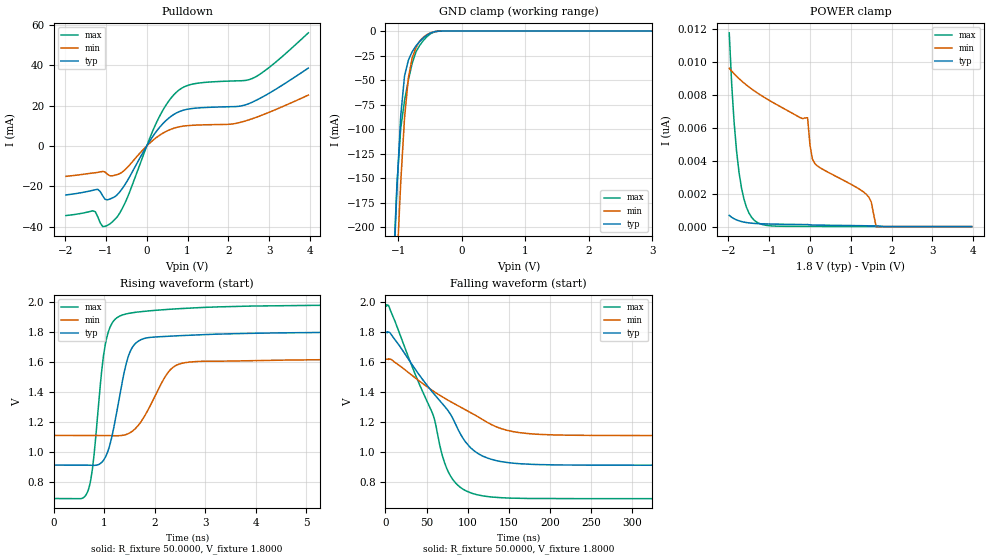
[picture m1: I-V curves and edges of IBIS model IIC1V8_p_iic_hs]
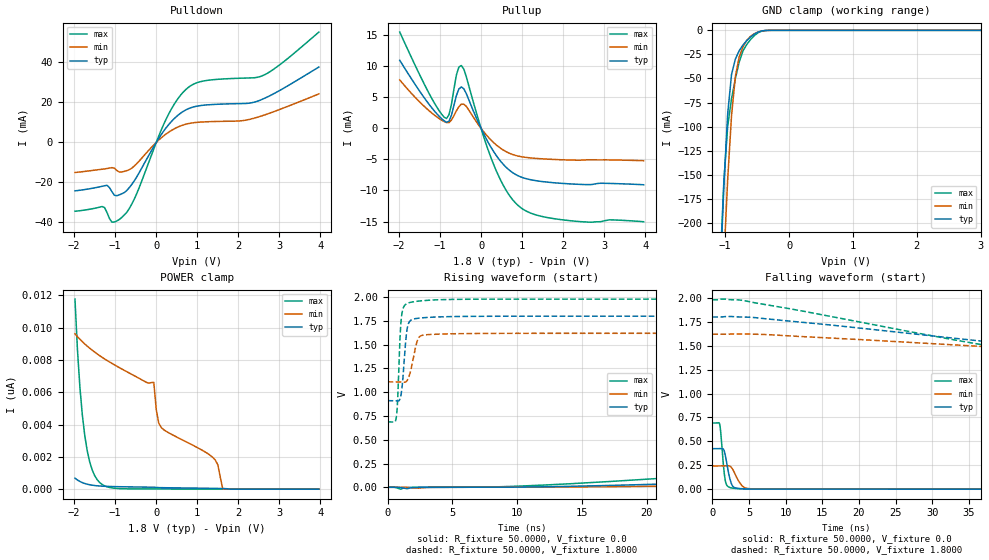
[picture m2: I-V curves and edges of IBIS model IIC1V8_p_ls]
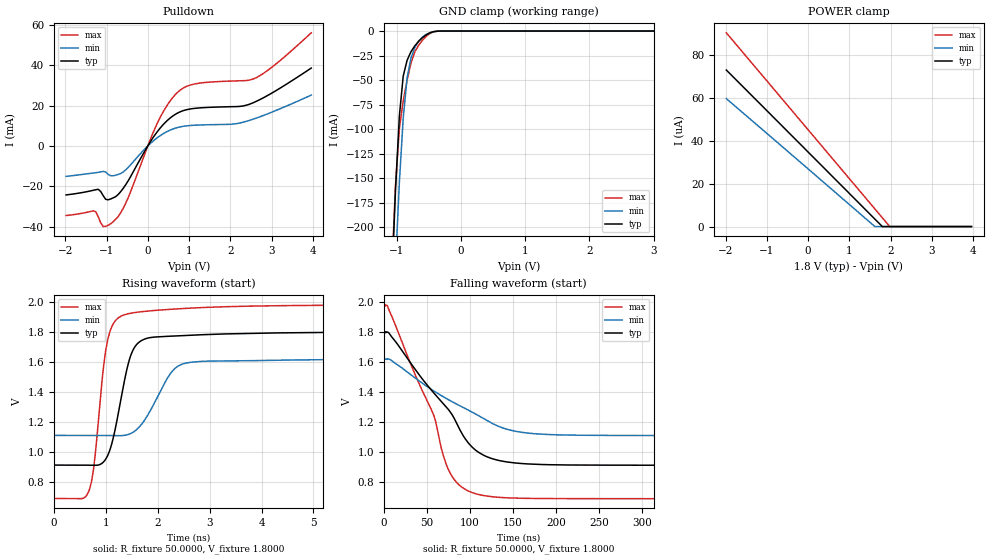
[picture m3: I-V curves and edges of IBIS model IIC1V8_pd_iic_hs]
| IBIS file qfp64afe_1p8v.ibs generated by Viper version: 2020.12.17
[IBIS Ver]   5.0
[Comment Char]   |_char
[File Name]   qfp64afe_1p8v.ibs
[File Rev]   1.3
[Date]   Thu Dec 17 17:50:21 2020
[Source]   NXP Viper 2020.12.17
[Notes]
[Disclaimer] IMPORTANT NOTICE
  This information is provided on an AS IS basis and without warranty.
  IN NO EVENT SHALL NXP BE LIABLE FOR INCIDENTAL OR CONSEQUENTIAL
  DAMAGES ARISING FROM USE OF THIS INFORMATION. THIS DISCLAIMER OF
  WARRANTY EXTENDS TO THE USER OF THE INFORMATION, AND TO THEIR CUSTOMERS
  OR USERS OF PRODUCTS  AND IS IN LIEU OF ALL WARRANTIES WHETHER EXPRESS,
  IMPLIED, OR STATUTORY, INCLUDING IMPLIED WARRANTIES OF MERCHANTABILITY
  OR FITNESS FOR PARTICULAR PURPOSE.
  NXP does not represent or warrant that the information furnished
  hereunder is free of infringement of any third party patents,
  copyrights, trade secrets, or other intellectual property rights.
  NXP does not represent or warrant that the information is free of
  defect, or that it meets any particular standard, requirements or need
  of the user of the infomation or their customers.
  NXP reserves the right to change the information in this file
  without notice.
   http://www.nxp.com
[Copyright]   (C) Copyright NXP 2004 - 2020, All Rights Reserved.
|   qfp64Afe
[Component]   qfp64Afe
[Manufacturer]   NXP
[Package]
| variable   typ   min   max
R_pkg   0.18002   0.098036   0.22836
L_pkg   3.270e-09   2.478e-09   3.882e-09
C_pkg   4.877e-13   4.194e-13   6.388e-13
[Pin] signal_name   model_name   R_pin   L_pin   C_pin
1   P2_1   gpio   0.20176   3.768e-09 4.934e-13
2   OPAMP2_INN   NC   0.18655   3.432e-09 5.614e-13
3   P0_1   gpio   0.1882   3.425e-09 5.543e-13
4   P1_0   gpio   0.18167   3.391e-09 4.852e-13
5   ADC1IN1B   NC   0.17508   3.272e-09 4.734e-13
6   ADC1IN1A   NC   0.17211   3.184e-09 4.709e-13
7   P0_11   gpio   0.17322   3.095e-09 4.516e-13
8   VDDA   POWER   NA   NA   NA
9   VREF_OUT   NC   0.098933  2.478e-09 5.107e-13
10   VREFP   NC   0.098036  2.682e-09 4.989e-13
11   VREFN   NC   0.10339   2.593e-09 5.200e-13
12   VSSA   GND   NA   NA   NA
13   P0_16   gpio   0.18219   3.272e-09 4.683e-13
14   P0_10   gpio   0.18473   3.372e-09 4.943e-13
15   P0_15   gpio   0.1948   3.518e-09 5.647e-13
16   P0_31   gpio   0.21166   3.882e-09 5.047e-13
17   P0_8   gpio   0.19981   3.690e-09 4.818e-13
18   OPAMP0_INN   NC   0.18485   3.354e-09 5.404e-13
19   P0_27   gpio   0.1771   3.251e-09 5.158e-13
20   OPAMP1_INN   NC   0.17264   3.242e-09 4.518e-13
21   XTAL32M_N   NC   0.17308   3.207e-09 4.514e-13
22   XTAL32M_P   NC   0.17099   3.143e-09 4.435e-13
23   RESETN   gpio   0.17312   3.058e-09 4.290e-13
24   VDD_CORE   POWER   NA   NA   NA
25   P1_22   gpio   0.17347   2.976e-09 4.359e-13
26   P0_17   gpio   0.17222   3.063e-09 4.368e-13
27   P0_7   gpio   0.17974   2.960e-09 4.541e-13
28   VDDE_2   POWER   NA   NA   NA
29   VSS_MAIN_PWR   GND   NA   NA   NA
30   VSS_MAIN   GND   NA   NA   NA
31   LX   NC   0.12471   2.527e-09 6.388e-13
32   VDD_MAIN_PWR   NC   NA   NA   NA
33   XTAL32K_P   NC   0.20305   3.722e-09 4.831e-13
34   XTAL32K_N   NC   0.18797   3.388e-09 5.425e-13
35   VBAT   NC   0.17937   3.272e-09 4.763e-13
36   P0_0   gpio   0.17575   3.216e-09 4.542e-13
37   P0_9   gpio   0.17142   3.151e-09 4.522e-13
38   P0_18   gpio   0.17027   3.108e-09 4.408e-13
39   P1_13   gpio   0.17092   3.083e-09 4.194e-13
40   P1_1   gpio   0.17351   3.079e-09 4.367e-13
41   P0_26   gpio   0.17937   3.140e-09 4.480e-13
42   P1_2   gpio   0.18924   3.260e-09 4.417e-13
43   P1_3   gpio   0.20575   3.278e-09 4.623e-13
44   VDDE_4   POWER   NA   NA   NA
45   P0_24   gpio   0.18768   3.277e-09 4.591e-13
46   P0_13   iic   0.19613   3.445e-09 5.506e-13
47   P0_14   iic   0.20782   3.616e-09 5.657e-13
48   P0_20   gpio   0.21594   3.876e-09 4.850e-13
49   P0_21   gpio   0.20723   3.837e-09 4.904e-13
50   P0_22   gpio   0.1962   3.547e-09 5.661e-13
51   P0_25   gpio   0.18792   3.420e-09 5.062e-13
52   P0_2   gpio   0.18663   3.397e-09 4.750e-13
53   P1_15   gpio   0.17882   3.273e-09 4.700e-13
54   P0_19   gpio   0.17446   3.156e-09 4.633e-13
55   P0_3   gpio   0.17673   3.008e-09 4.457e-13
56   VDDE_4   POWER   NA   NA   NA
57   P0_4   gpio   0.17637   3.003e-09 4.457e-13
58   P1_16   gpio   0.17537   3.170e-09 4.476e-13
59   P0_6   gpio   0.17935   3.248e-09 4.687e-13
60   P0_5   gpio   0.18758   3.378e-09 4.757e-13
61   P0_29   gpio   0.19171   3.430e-09 4.834e-13
62   P1_11   gpio   0.20582   3.539e-09 5.647e-13
63   P0_30   gpio   0.22836   3.428e-09 5.818e-13
64   VDDE_4   POWER   NA   NA   NA
65   VSS   GND   NA   NA   NA
[Pin Mapping]   pulldown_ref   pullup_ref
1   VSS   VDDA
2   NC   NC
3   VSS   VDDA
4   VSS   VDDA
5   NC   NC
6   NC   NC
7   VSS   VDDA
8   NC   VDDA
9   NC   NC
10   NC   NC
11   NC   NC
12   VSSA   NC
13   VSS   VDDA
14   VSS   VDDA
15   VSS   VDDA
16   VSS   VDDA
17   VSS   VDDA
18   NC   NC
19   VSS   VDDA
20   NC   NC
21   NC   NC
22   NC   NC
23   VSS   VDDE_2
24   NC   VDD_CORE
25   VSS   VDDE_2
26   VSS   VDDE_2
27   VSS   VDDE_2
28   NC   VDDE_2
29   VSS_MAIN_PWR   NC
30   VSS_MAIN   NC
31   NC   NC
32   NC   NC
33   NC   NC
34   NC   NC
35   NC   NC
36   VSS   VDDE_4
37   VSS   VDDE_4
38   VSS   VDDE_4
39   VSS   VDDE_4
40   VSS   VDDE_4
41   VSS   VDDE_4
42   VSS   VDDE_4
43   VSS   VDDE_4
44   NC   VDDE_4
45   VSS   VDDE_4
46   VSS   VDDE_4
47   VSS   VDDE_4
48   VSS   VDDE_4
49   VSS   VDDE_4
50   VSS   VDDE_4
51   VSS   VDDE_4
52   VSS   VDDE_4
53   VSS   VDDE_4
54   VSS   VDDE_4
55   VSS   VDDE_4
56   NC   VDDE_4
57   VSS   VDDE_4
58   VSS   VDDE_4
59   VSS   VDDE_4
60   VSS   VDDE_4
61   VSS   VDDE_4
62   VSS   VDDE_4
63   VSS   VDDE_4
64   NC   VDDE_4
65   VSS   NC
|*   Model Selector   *
[Model Selector] gpio
MFIO1V8_pd_hs   EPUN=1 EPD=1 EHS=1
MFIO1V8_pd_ls   EPUN=1 EPD=1 EHS=0
MFIO1V8_pu_hs   EPUN=0 EPD=0 EHS=1
MFIO1V8_pu_ls   EPUN=0 EPD=0 EHS=0
MFIO1V8_p_hs   EPUN=1 EPD=0 EHS=1
MFIO1V8_p_ls   EPUN=1 EPD=0 EHS=0
MFIO1V8_r_hs   EPUN=0 EPD=1 EHS=1
MFIO1V8_r_ls   EPUN=0 EPD=1 EHS=0
[Model Selector] iic
IIC1V8_pd_hs   EGP=1 EPUN=1 EPD=1 EHS=1
IIC1V8_pd_ls   EGP=1 EPUN=1 EPD=1 EHS=0
IIC1V8_p_hs   EGP=1 EPUN=1 EPD=0 EHS=1
IIC1V8_p_ls   EGP=1 EPUN=1 EPD=0 EHS=0
IIC1V8_pu_hs   EGP=1 EPUN=0 EPD=0 EHS=1
IIC1V8_pu_ls   EGP=1 EPUN=0 EPD=0 EHS=0
IIC1V8_r_hs   EGP=1 EPUN=0 EPD=1 EHS=1
IIC1V8_r_ls   EGP=1 EPUN=0 EPD=1 EHS=0
IIC1V8_pd_iic_hs   EGP=0 ECS=0 EPUN=1 EPD=1
IIC1V8_p_iic_hs   EGP=0 ECS=0 EPUN=1 EPD=0
IIC1V8_pu_iic_hs   EGP=0 ECS=0 EPUN=0 EPD=0
IIC1V8_r_iic_hs   EGP=0 ECS=0 EPUN=0 EPD=1
IIC1V8_pd_iic_pu_hs   EGP=0 ECS=1 EPUN=1 EPD=1 SSEL=1
IIC1V8_p_iic_pu_hs   EGP=0 ECS=1 EPUN=1 EPD=0 SSEL=1
IIC1V8_pu_iic_pu_hs   EGP=0 ECS=1 EPUN=0 EPD=0 SSEL=1
IIC1V8_r_iic_pu_hs   EGP=0 ECS=1 EPUN=0 EPD=1 SSEL=1
| End [Component] qfp64Afe
| Models and submodels in the file (24): IIC1V8_p_hs (I/O), IIC1V8_p_iic_hs (I/O_open_drain), IIC1V8_p_iic_pu_hs (I/O_open_drain), IIC1V8_p_ls (I/O), IIC1V8_pd_hs (I/O), IIC1V8_pd_iic_hs (I/O_open_drain), IIC1V8_pd_iic_pu_hs (I/O_open_drain), IIC1V8_pd_ls (I/O), IIC1V8_pu_hs (I/O), IIC1V8_pu_iic_hs (I/O_open_drain), IIC1V8_pu_iic_pu_hs (I/O_open_drain), IIC1V8_pu_ls (I/O), IIC1V8_r_hs (I/O), IIC1V8_r_iic_hs (I/O_open_drain), IIC1V8_r_iic_pu_hs (I/O_open_drain), IIC1V8_r_ls (I/O), MFIO1V8_p_hs (I/O), MFIO1V8_p_ls (I/O), MFIO1V8_pd_hs (I/O), MFIO1V8_pd_ls (I/O), MFIO1V8_pu_hs (I/O), MFIO1V8_pu_ls (I/O), MFIO1V8_r_hs (I/O), MFIO1V8_r_ls (I/O)
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[Model] IIC1V8_p_iic_hs
|   Model IIC1V8_p_iic_hs
| This model was characterised for following simulation conditions:
| External (pad) voltage:
|   - Typ: 1.8V,   - Min: 1.62V,   - Max: 1.98V
| Library cells for typ/min/max conditions are connected as defined below:
|  IO - External Pad
|  A - Core Input
|  EN - Output Buffer Enable
|  BOOST - vdde
|  ECS - gnd
|  EGP - gnd
|  ENZI - vdd
|  EPD - gnd
|  EPUN - vdd
|  ZI - NC
|  ZIF - NC
|  gnd - gnd
|  gnde - gnde
|  vdd - vdd
|  vdde - vdde
| All other pins connected to ground
Model_type I/O_open_drain
Polarity   Non-Inverting
Enable   Active-Low
Vinl =   0.5400V
Vinh =   1.2600V
Vmeas =  0.9000V
Cref =   0.0F
Rref =   1000.000
Vref =   1.8000V
C_comp   3.6454pF   3.5038pF   3.7808pF
|C_comp_pullup   0.9524pF   0.9269pF   0.9624pF
|C_comp_pulldown   2.3410pF   2.4924pF   2.1971pF
[Model Spec]
| variable   typ   min   max
Vinh   0.5400V   0.4860V   0.5940V
Vinl   1.2600V   1.1340V   1.3860V
Vmeas   0.9000V   0.8100V   0.9900V
Vref   1.8000V   1.6200V   1.9800V
Cref   0.0F   0.0F   0.0F
Rref   1.0000k   1.0000k   1.0000k
[Temperature Range]   25.0000   0.1250k   -40.0000
[Voltage Range]   1.8000V   1.6200V   1.9800V
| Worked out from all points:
|   slope of the pulldown table from 0 to 0.27 V, typ, clamps not added: 33.4 ohm
|   GND clamp passes 1 mA (typ) near -0.44 V on its own axis
|   rising waveform, R_fixture 50.0000, V_fixture 1.8000: 20-80 % time 321ps typ, 491ps min, 237ps max; typ from 0.911 V to 1.8 V
|   falling waveform, R_fixture 50.0000, V_fixture 1.8000: 20-80 % time 66.9ns typ, 88.7ns min, 48.9ns max; typ from 1.8 V to 0.911 V
[Pulldown]
|Voltage   I(typ)   I(min)   I(max)
-1.98V    -24.22mA   -15.04mA   -34.42mA
-1.32V    -21.94mA   -13.4mA    -32.06mA
-1.2V     -21.45mA   -13.05mA   -35.06mA
-1.08V    -24.63mA   -12.6mA    -39.9mA
-900mV    -26.23mA   -14.78mA   -38.53mA
-540mV    -19.33mA   -11.9mA    -28.53mA
300mV     8.856mA    5.096mA    14.12mA
720mV     16.26mA    9.117mA    26.48mA
1.14V     18.6mA     10.26mA    30.69mA
2.1V      19.45mA    10.9mA     32.16mA
2.58V     21.61mA    13.44mA    33.34mA
3.96V     38.56mA    25.19mA    55.99mA
[GND_clamp]
|Voltage   I(typ)   I(min)   I(max)
-1.98V    -2.104A    -2.075A    -2.136A
-1.08V    -259.3mA   -333mA     -246.9mA
-1.02V    -161.8mA   -238.7mA   -157.1mA
-960mV    -86.74mA   -154.7mA   -99.46mA
-900mV    -45.95mA   -88.82mA   -71.05mA
-840mV    -29.9mA    -47.99mA   -50.25mA
-780mV    -21.15mA   -27.64mA   -32.98mA
-720mV    -15.16mA   -16.87mA   -21.26mA
-660mV    -10.56mA   -10.24mA   -14.56mA
-540mV    -3.788mA   -3.398mA   -5.292mA
-300mV    -15.94uA   -36uA      -16.34uA
3.96V     0A         0A         0A
[POWER_clamp]
|Voltage   I(typ)   I(min)   I(max)
-1.98V    679.6pA    9.61nA     11.76nA
-1.86V    475.2pA    9.277nA    6.313nA
-1.74V    349.2pA    8.982nA    3.292nA
-1.56V    245.6pA    8.597nA    1.186nA
-1.32V    186pA      8.161nA    293.2pA
-60mV     124.8pA    6.606nA    14.31pA
0V        105.5pA    4.916nA    11.81pA
120mV     93.21pA    3.82nA     10.91pA
1.38V     50pA       1.96nA     2.877pA
1.5V      45.28pA    1.501nA    2.149pA
1.62V     39.18pA    0A         1.42pA
3.96V     0A         0A         0A
[Ramp]
| variable   typ   min   max
dV/dt_r  0.5334/0.3209n   0.3066/0.4909n   0.7753/0.2369n
dV/dt_f  0.5334/66.9323n   0.3066/88.7325n   0.7753/48.9497n
R_load = 50.0000
[Rising Waveform]
R_fixture= 50.0000
V_fixture= 1.8000
V_fixture_min= 1.6200
V_fixture_max= 1.9800
|time   V(typ)   V(min)   V(max)
0s        911mV      1.109V     687.8mV
683.3ps   910.2mV    1.109V     745.5mV
780.5ps   909.1mV    1.109V     927.7mV
1.017ns   961.1mV    1.108V     1.71V
1.277ns   1.32V      1.107V     1.9V
1.506ns   1.663V     1.126V     1.925V
1.797ns   1.757V     1.237V     1.938V
2.547ns   1.776V     1.591V     1.956V
6.124ns   1.798V     1.616V     1.979V
1us       1.8V       1.62V      1.98V
[Falling Waveform]
R_fixture= 50.0000
V_fixture= 1.8000
V_fixture_min= 1.6200
V_fixture_max= 1.9800
|time   V(typ)   V(min)   V(max)
0s        1.8V       1.62V      1.98V
4.033ns   1.8V       1.621V     1.975V
57.1ns    1.4V       1.41V      1.258V
68.97ns   1.323V     1.369V     978.6mV
76.93ns   1.269V     1.343V     860.5mV
95.01ns   1.085V     1.288V     749mV
110.3ns   997.3mV    1.242V     715.6mV
148.2ns   929.5mV    1.144V     692.6mV
208ns     913.4mV    1.113V     688.4mV
1us       911.1mV    1.109V     687.9mV
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[Model] IIC1V8_p_ls
|   Model IIC1V8_p_ls
| This model was characterised for following simulation conditions:
| External (pad) voltage:
|   - Typ: 1.8V,   - Min: 1.62V,   - Max: 1.98V
| Library cells for typ/min/max conditions are connected as defined below:
|  IO - External Pad
|  A - Core Input
|  EN - Output Buffer Enable
|  BOOST - vdde
|  EGP - vdd
|  EHS - gnd
|  ENZI - vdd
|  EPD - gnd
|  EPUN - vdd
|  ZI - NC
|  ZIF - NC
|  gnd - gnd
|  gnde - gnde
|  vdd - vdd
|  vdde - vdde
| All other pins connected to ground
Model_type I/O
Polarity   Non-Inverting
Enable   Active-Low
Vinl =   0.5400V
Vinh =   1.2600V
Vmeas =  0.9000V
Cref =   0.0F
Rref =   1.0000k
Vref =   0.0V
C_comp   3.6452pF   3.5037pF   3.7805pF
|C_comp_pullup   0.9521pF   0.9262pF   0.9623pF
|C_comp_pulldown   2.3411pF   2.4927pF   2.1971pF
[Model Spec]
| variable   typ   min   max
Vinh   0.5400V   0.4860V   0.5940V
Vinl   1.2600V   1.1340V   1.3860V
Vmeas   0.9000V   0.8100V   0.9900V
[Temperature Range]   25.0000   0.1250k   -40.0000
[Voltage Range]   1.8000V   1.6200V   1.9800V
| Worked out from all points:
|   slope of the pulldown table from 0 to 0.27 V, typ, clamps not added: 33.4 ohm
|   slope of the pullup table from 0 to 0.27 V, typ, clamps not added: 80.7 ohm
|   GND clamp passes 1 mA (typ) near -0.44 V on its own axis
|   rising waveform, R_fixture 50.0000, V_fixture 0.0: 20-80 % time 70.1ns typ, 82ns min, 57.1ns max; typ from 0 V to 0.423 V
|   rising waveform, R_fixture 50.0000, V_fixture 1.8000: 20-80 % time 319ps typ, 487ps min, 235ps max; typ from 0.911 V to 1.8 V
|   falling waveform, R_fixture 50.0000, V_fixture 0.0: 20-80 % time 672ps typ, 1.04ns min, 474ps max; typ from 0.423 V to 0 V
|   falling waveform, R_fixture 50.0000, V_fixture 1.8000: 20-80 % time 66.9ns typ, 88.7ns min, 49ns max; typ from 1.8 V to 0.911 V
[Pulldown]
|Voltage   I(typ)   I(min)   I(max)
-1.98V    -24.22mA   -15.04mA   -34.42mA
-1.32V    -21.94mA   -13.4mA    -32.06mA
-1.2V     -21.45mA   -13.05mA   -35.06mA
-1.08V    -24.63mA   -12.6mA    -39.9mA
-900mV    -26.23mA   -14.78mA   -38.53mA
-720mV    -24.07mA   -14.13mA   -34.99mA
-540mV    -19.33mA   -11.9mA    -28.53mA
300mV     8.856mA    5.096mA    14.12mA
720mV     16.26mA    9.117mA    26.48mA
1.14V     18.6mA     10.26mA    30.69mA
2.58V     21.56mA    13.35mA    33.32mA
3.96V     37.73mA    24.28mA    55.2mA
[Pullup]
|Voltage   I(typ)   I(min)   I(max)
-1.98V    10.95mA    7.799mA    15.5mA
-1.32V    4.346mA    3.159mA    6.304mA
-900mV    1.218mA    1.094mA    1.804mA
-780mV    1.156mA    929.2uA    2.224mA
-600mV    5.286mA    2.831mA    8.611mA
-480mV    6.667mA    3.906mA    10.12mA
-420mV    6.372mA    3.889mA    9.539mA
360mV     -4.265mA   -2.608mA   -6.666mA
660mV     -6.57mA    -3.917mA   -10.5mA
960mV     -7.8mA     -4.537mA   -12.74mA
2.04V     -8.889mA   -5.075mA   -14.77mA
3.96V     -9.081mA   -5.209mA   -15.04mA
[GND_clamp]
|Voltage   I(typ)   I(min)   I(max)
-1.98V    -2.104A    -2.075A    -2.136A
-1.08V    -259.3mA   -333mA     -246.9mA
-1.02V    -161.8mA   -238.7mA   -157.1mA
-960mV    -86.74mA   -154.7mA   -99.46mA
-900mV    -45.95mA   -88.82mA   -71.05mA
-840mV    -29.9mA    -47.99mA   -50.25mA
-780mV    -21.15mA   -27.64mA   -32.98mA
-720mV    -15.16mA   -16.87mA   -21.26mA
-660mV    -10.56mA   -10.24mA   -14.56mA
-540mV    -3.788mA   -3.398mA   -5.292mA
-300mV    -15.94uA   -36uA      -16.34uA
3.96V     0A         0A         0A
[POWER_clamp]
|Voltage   I(typ)   I(min)   I(max)
-1.98V    679.6pA    9.61nA     11.76nA
-1.86V    475.2pA    9.277nA    6.313nA
-1.74V    349.2pA    8.982nA    3.292nA
-1.56V    245.6pA    8.597nA    1.186nA
-1.32V    186pA      8.161nA    293.2pA
-60mV     124.8pA    6.606nA    14.31pA
0V        105.5pA    4.916nA    11.81pA
120mV     93.21pA    3.82nA     10.91pA
1.38V     50pA       1.96nA     2.877pA
1.5V      45.28pA    1.501nA    2.149pA
1.62V     39.18pA    0A         1.42pA
3.96V     0A         0A         0A
[Ramp]
| variable   typ   min   max
dV/dt_r  0.2539/70.1178n   0.1457/81.9302n   0.4150/57.0489n
dV/dt_f  0.5334/66.9358n   0.3066/88.6649n   0.7753/48.9538n
R_load = 50.0000
[Rising Waveform]
R_fixture= 50.0000
V_fixture= 0.0
V_fixture_min= 0.0
V_fixture_max= 0.0
|time   V(typ)   V(min)   V(max)
0s        602.8pV    52.95nV    41.9pV
1.012ns   -3.31mV    192.5uV    -19.98mV
1.632ns   -11.39mV   -2.738mV   -1.795mV
12.68ns   6.299mV    1.388mV    27.19mV
45.88ns   145.4mV    64.89mV    304.8mV
84.55ns   285.2mV    143.4mV    561.1mV
103.3ns   339.8mV    172mV      629.2mV
134ns     392.1mV    207.9mV    672.5mV
250.9ns   422.4mV    241.3mV    691.3mV
1us       423.2mV    242.8mV    691.7mV
[Rising Waveform]
R_fixture= 50.0000
V_fixture= 1.8000
V_fixture_min= 1.6200
V_fixture_max= 1.9800
|time   V(typ)   V(min)   V(max)
0s        911mV      1.109V     687.8mV
685.2ps   909.5mV    1.109V     745.1mV
787ps     907.1mV    1.109V     945.8mV
1.007ns   951.3mV    1.108V     1.694V
1.269ns   1.304V     1.105V     1.904V
1.479ns   1.639V     1.118V     1.932V
1.768ns   1.755V     1.218V     1.945V
2.476ns   1.78V      1.585V     1.96V
5.596ns   1.797V     1.616V     1.978V
1us       1.8V       1.62V      1.98V
[Falling Waveform]
R_fixture= 50.0000
V_fixture= 0.0
V_fixture_min= 0.0
V_fixture_max= 0.0
|time   V(typ)   V(min)   V(max)
0s        423.2mV    242.8mV    691.7mV
1.011ns   423.2mV    242.8mV    674.4mV
1.154ns   424.5mV    242.8mV    586.3mV
1.621ns   398.5mV    242.8mV    166.3mV
1.942ns   280.1mV    244.4mV    44.84mV
2.413ns   102.2mV    239.4mV    16.8mV
2.833ns   25.91mV    200.2mV    9.661mV
4.004ns   4.701mV    40.3mV     3.498mV
5.055ns   2.01mV     5.162mV    2.038mV
1us       19.02nV    85.51nV    10.92nV
[Falling Waveform]
R_fixture= 50.0000
V_fixture= 1.8000
V_fixture_min= 1.6200
V_fixture_max= 1.9800
|time   V(typ)   V(min)   V(max)
0s        1.8V       1.62V      1.98V
4.079ns   1.8V       1.623V     1.975V
57.22ns   1.399V     1.41V      1.256V
69.33ns   1.321V     1.367V     971.7mV
77.23ns   1.267V     1.342V     857.4mV
95.69ns   1.079V     1.287V     746.9mV
111ns     994.9mV    1.239V     714.6mV
149.1ns   928.8mV    1.143V     692.4mV
207.1ns   913.6mV    1.113V     688.4mV
1us       911.1mV    1.109V     687.9mV
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[Model] IIC1V8_pd_iic_hs
|   Model IIC1V8_pd_iic_hs
| This model was characterised for following simulation conditions:
| External (pad) voltage:
|   - Typ: 1.8V,   - Min: 1.62V,   - Max: 1.98V
| Library cells for typ/min/max conditions are connected as defined below:
|  IO - External Pad
|  A - Core Input
|  EN - Output Buffer Enable
|  BOOST - vdde
|  ECS - gnd
|  EGP - gnd
|  ENZI - vdd
|  EPD - vdd
|  EPUN - vdd
|  ZI - NC
|  ZIF - NC
|  gnd - gnd
|  gnde - gnde
|  vdd - vdd
|  vdde - vdde
| All other pins connected to ground
Model_type I/O_open_drain
Polarity   Non-Inverting
Enable   Active-Low
Vinl =   0.5400V
Vinh =   1.2600V
Vmeas =  0.9000V
Cref =   0.0F
Rref =   1000.000
Vref =   1.8000V
C_comp   3.6138pF   3.4666pF   3.7547pF
|C_comp_pullup   0.9378pF   0.9163pF   0.9441pF
|C_comp_pulldown   2.3253pF   2.4781pF   2.1797pF
[Model Spec]
| variable   typ   min   max
Vinh   0.5400V   0.4860V   0.5940V
Vinl   1.2600V   1.1340V   1.3860V
Vmeas   0.9000V   0.8100V   0.9900V
Vref   1.8000V   1.6200V   1.9800V
Cref   0.0F   0.0F   0.0F
Rref   1.0000k   1.0000k   1.0000k
[Temperature Range]   25.0000   0.1250k   -40.0000
[Voltage Range]   1.8000V   1.6200V   1.9800V
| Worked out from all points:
|   slope of the pulldown table from 0 to 0.27 V, typ, clamps not added: 33.4 ohm
|   GND clamp passes 1 mA (typ) near -0.44 V on its own axis
|   rising waveform, R_fixture 50.0000, V_fixture 1.8000: 20-80 % time 320ps typ, 490ps min, 236ps max; typ from 0.91 V to 1.8 V
|   falling waveform, R_fixture 50.0000, V_fixture 1.8000: 20-80 % time 66.8ns typ, 88.6ns min, 48.9ns max; typ from 1.8 V to 0.91 V
[Pulldown]
|Voltage   I(typ)   I(min)   I(max)
-1.98V    -24.22mA   -15.04mA   -34.42mA
-1.32V    -21.94mA   -13.4mA    -32.06mA
-1.2V     -21.45mA   -13.05mA   -35.06mA
-1.08V    -24.63mA   -12.6mA    -39.9mA
-900mV    -26.23mA   -14.78mA   -38.53mA
-540mV    -19.33mA   -11.9mA    -28.53mA
300mV     8.856mA    5.096mA    14.12mA
720mV     16.26mA    9.117mA    26.48mA
1.14V     18.6mA     10.26mA    30.69mA
2.1V      19.45mA    10.89mA    32.16mA
2.58V     21.61mA    13.43mA    33.34mA
3.96V     38.53mA    25.17mA    55.97mA
[GND_clamp]
|Voltage   I(typ)   I(min)   I(max)
-1.98V    -2.104A    -2.075A    -2.136A
-1.08V    -259.3mA   -333mA     -246.9mA
-1.02V    -161.8mA   -238.7mA   -157.1mA
-960mV    -86.75mA   -154.7mA   -99.47mA
-900mV    -45.96mA   -88.82mA   -71.06mA
-840mV    -29.91mA   -48mA      -50.26mA
-780mV    -21.16mA   -27.65mA   -32.99mA
-720mV    -15.17mA   -16.88mA   -21.27mA
-660mV    -10.57mA   -10.24mA   -14.57mA
-540mV    -3.796mA   -3.405mA   -5.301mA
-300mV    -21.69uA   -40.85uA   -23.15uA
3.96V     0A         0A         0A
[POWER_clamp]
|Voltage   I(typ)   I(min)   I(max)
-1.98V    73.06uA    59.72uA    90.42uA
1.62V     3.484uA    0A         8.225uA
1.8V      0A         0A         4.113uA
1.98V     0A         0A         0A
3.96V     0A         0A         0A
[Ramp]
| variable   typ   min   max
dV/dt_r  0.5328/0.3204n   0.3064/0.4905n   0.7742/0.2363n
dV/dt_f  0.5327/66.8167n   0.3063/88.5485n   0.7742/48.8803n
R_load = 50.0000
[Rising Waveform]
R_fixture= 50.0000
V_fixture= 1.8000
V_fixture_min= 1.6200
V_fixture_max= 1.9800
|time   V(typ)   V(min)   V(max)
0s        910.3mV    1.108V     687.5mV
683.8ps   909.5mV    1.108V     745.6mV
781ps     908.4mV    1.108V     928.7mV
1.004ns   952.7mV    1.108V     1.684V
1.256ns   1.281V     1.106V     1.895V
1.48ns    1.64V      1.121V     1.922V
1.782ns   1.754V     1.228V     1.936V
2.499ns   1.774V     1.586V     1.954V
5.711ns   1.796V     1.614V     1.976V
1us       1.798V     1.619V     1.978V
[Falling Waveform]
R_fixture= 50.0000
V_fixture= 1.8000
V_fixture_min= 1.6200
V_fixture_max= 1.9800
|time   V(typ)   V(min)   V(max)
0s        1.798V     1.619V     1.978V
4.099ns   1.798V     1.62V      1.972V
58.16ns   1.391V     1.405V     1.24V
68.8ns    1.323V     1.368V     979.5mV
76.88ns   1.268V     1.342V     859.4mV
94.48ns   1.087V     1.289V     749.9mV
110.4ns   995.3mV    1.24V      714.9mV
145.3ns   930.8mV    1.147V     692.8mV
202.8ns   913.2mV    1.113V     688.1mV
1us       910.4mV    1.108V     687.5mV
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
